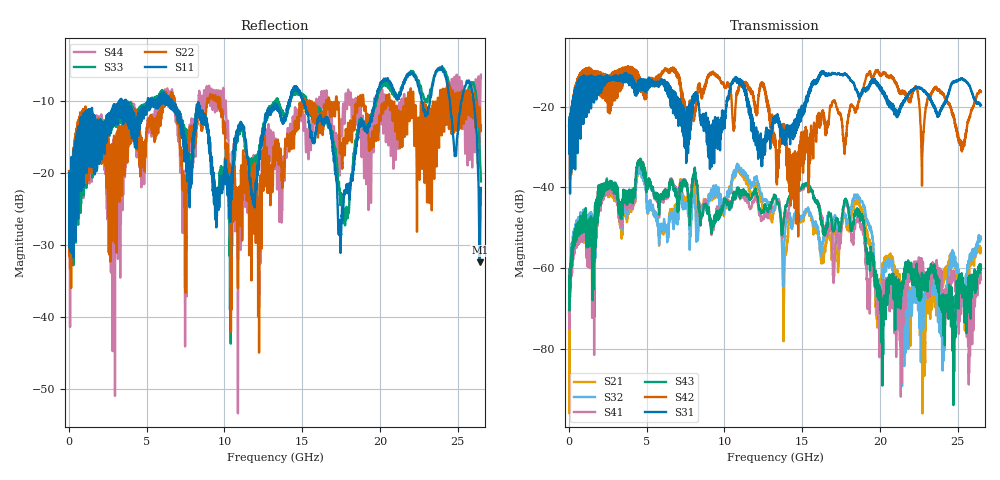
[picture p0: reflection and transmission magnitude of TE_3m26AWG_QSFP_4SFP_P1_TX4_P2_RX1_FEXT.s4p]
!Agilent Technologies,N5222A,MY51421691,A.10.00.00
!Agilent N5222A: A.10.00.00
!Date: Friday, January 30, 2015 12:37:33
!Correction: S11(Full 4 Port(1,2,3,4))
!S12(Full 4 Port(1,2,3,4))
!S13(Full 4 Port(1,2,3,4))
!S14(Full 4 Port(1,2,3,4))
!S21(Full 4 Port(1,2,3,4))
!S22(Full 4 Port(1,2,3,4))
!S23(Full 4 Port(1,2,3,4))
!S24(Full 4 Port(1,2,3,4))
!S31(Full 4 Port(1,2,3,4))
!S32(Full 4 Port(1,2,3,4))
!S33(Full 4 Port(1,2,3,4))
!S34(Full 4 Port(1,2,3,4))
!S41(Full 4 Port(1,2,3,4))
!S42(Full 4 Port(1,2,3,4))
!S43(Full 4 Port(1,2,3,4))
!S44(Full 4 Port(1,2,3,4))
!S4P File: Measurements: <S11,S12,S13,S14>,
!<S21,S22,S23,S24>,
!<S31,S32,S33,S34>,
!<S41,S42,S43,S44>:
# Hz S  dB  R 50.0
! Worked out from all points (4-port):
!   2650 points, 10 MHz to 26.5 GHz, reference 50 ohm
!   strongest paths, dB at 10 MHz, 6.63 GHz, 13.26 GHz, 19.88 GHz, 26.5 GHz:
!     S31: -24.8, -19.0, -23.3, -14.9, -19.7
!     S42: -24.9, -11.2, -27.5, -11.3, -16.4
!     S43: -62.0, -38.2, -42.2, -65.1, -59.7
!     S41: -69.7, -38.1, -42.2, -67.8, -62.8
!     S32: -71.6, -46.3, -45.3, -69.1, -52.5
!     S21: -65.7, -45.7, -45.3, -64.4, -55.5
!   lowest |S11| = -32.4 dB at 26.43 GHz (marker M1), VSWR 1.05, Z = 51.8 - j1.59 ohm
!   |S11| at or under -10 dB: start of sweep to 3.24 GHz; 6.606 GHz to 14.16 GHz (7.55 GHz wide, 72.7 % of centre); 15.11 GHz to 19.68 GHz (4.573 GHz wide, 26.3 % of centre)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
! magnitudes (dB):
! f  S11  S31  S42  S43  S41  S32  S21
! 10 MHz  -20.0  -24.8  -24.9  -62.0  -69.7  -71.6  -65.7
! 4.54 GHz  -13.0  -13.6  -13.0  -34.2  -34.4  -36.3  -36.6
! 13.85 GHz  -12.5  -29.1  -25.1  -47.4  -47.8  -54.7  -61.5
! 18.51 GHz  -16.0  -15.8  -20.6  -46.3  -47.9  -42.6  -44.1
! 21.44 GHz  -8.0  -19.2  -16.7  -64.7  -73.5  -76.7  -64.7
! 26.43 GHz  -32.4  -19.4  -16.0  -59.5  -62.6  -52.4  -55.2
! 26.5 GHz  -22.1  -19.7  -16.4  -59.7  -62.8  -52.5  -55.5
